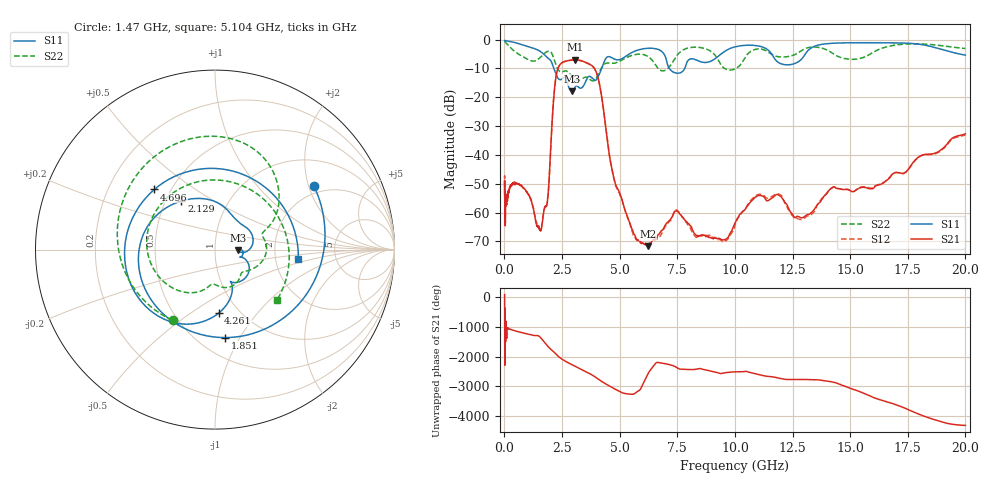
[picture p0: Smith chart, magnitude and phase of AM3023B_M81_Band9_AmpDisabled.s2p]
!Agilent Technologies,E8364B,MY43040894,A.07.50.67
!Agilent E8364B: A.07.50.67
!Date: Tuesday, October 27, 2020 10:40:56
!Correction: S11(Full 2 Port(1,2))
!S21(Full 2 Port(1,2))
!S12(Full 2 Port(1,2))
!S22(Full 2 Port(1,2))
!S2P File: Measurements: S11, S21, S12, S22:Log Frequency Sweep
# Hz S  dB  R 50
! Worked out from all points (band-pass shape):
!   3201 points, 10 MHz to 20 GHz, reference 50 ohm
!   highest |S21| = -7.00 dB at 3.07 GHz (marker M1); lowest = -71.7 dB at 6.231 GHz (marker M2)
!   |S21| within 3 dB of the highest: 2.323 GHz to 3.907 GHz (1.585 GHz wide, 50.9 % of centre)
!   lowest |S11| = -17.9 dB at 2.92 GHz (marker M3), VSWR 1.29, Z = 64.6 - j0.277 ohm
!   |S11| at or under -10 dB: 2.145 GHz to 4.213 GHz (2.068 GHz wide, 65 % of centre); 7.158 GHz to 7.825 GHz (667.3 MHz wide, 8.91 % of centre)
!   |S22| runs from -14.3 to -0.6 dB; largest |S21 - S12| = 0.0073
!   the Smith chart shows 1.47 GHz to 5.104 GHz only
!   S11 on the Smith chart (normalised r, x): 1.47 GHz: 1.75, +2.16; 1.851 GHz: 0.67, -0.87; 2.129 GHz: 0.60, +0.37; 4.261 GHz: 0.81, -0.65; 4.696 GHz: 0.41, +0.35; 5.104 GHz: 2.69, -0.38
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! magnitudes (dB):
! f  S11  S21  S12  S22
! 10 MHz  -0.3  -54.2  -51.2  -0.6
! 35.55 MHz  -0.4  -63.3  -62.8  -0.8
! 126.1 MHz  -0.5  -54.2  -54.8  -1.6
! 447.2 MHz  -1.0  -50.1  -49.6  -4.1
! 1.47 GHz  -3.7  -65.0  -64.6  -6.8
! 1.59 GHz  -4.3  -66.1  -66.0  -5.9
! 1.851 GHz  -6.1  -56.9  -57.2  -4.2
! 2.129 GHz  -9.6  -21.3  -21.4  -6.2
! 2.347 GHz  -13.6  -9.5  -9.6  -10.6
! 2.92 GHz  -17.9  -7.1  -7.1  -12.5
! 3.07 GHz  -16.5  -7.0  -7.1  -13.6
! 3.874 GHz  -13.8  -9.6  -9.7  -14.3
! 4.261 GHz  -9.0  -22.0  -22.0  -9.3
! 4.696 GHz  -6.4  -46.0  -46.2  -8.2
! 5.104 GHz  -6.6  -55.5  -55.6  -7.0
! 5.639 GHz  -4.1  -67.5  -68.2  -5.2
! 6.231 GHz  -3.0  -71.7  -71.3  -5.8
! 7.481 GHz  -11.6  -59.5  -59.1  -5.5
! 9.532 GHz  -4.2  -69.5  -70.1  -9.9
! 11.18 GHz  -2.5  -54.2  -53.8  -3.3
! 12.98 GHz  -5.9  -61.6  -62.1  -3.4
! 20 GHz  -5.4  -32.7  -33.1  -3.1
